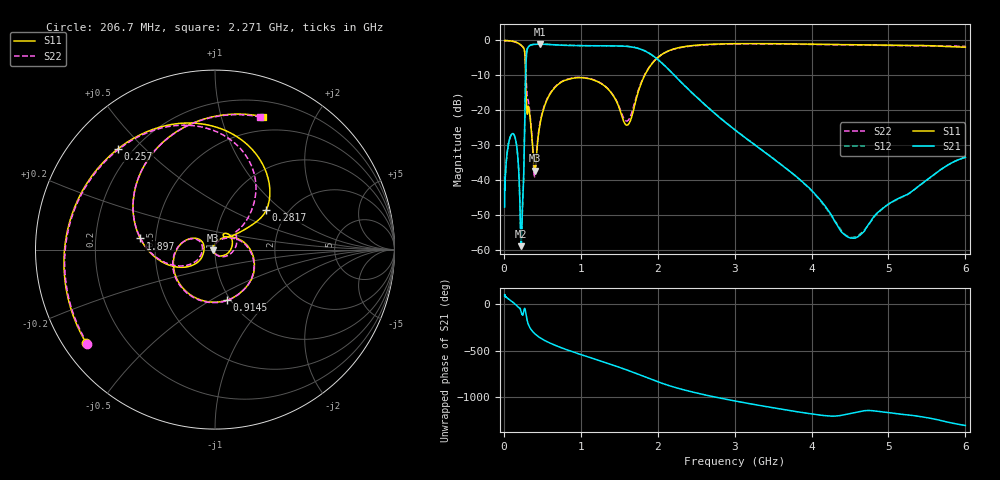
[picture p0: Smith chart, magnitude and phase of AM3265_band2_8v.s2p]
!Agilent Technologies,E8364B,MY43040894,A.07.50.67
!Agilent E8364B: A.07.50.67
!Date: Friday, May 09, 2025 07:26:20
!Correction: S11(Full 2 Port(1,2))
!S21(Full 2 Port(1,2))
!S12(Full 2 Port(1,2))
!S22(Full 2 Port(1,2))
!S2P File: Measurements: S11, S21, S12, S22:Log Frequency Sweep
# Hz S  dB  R 50
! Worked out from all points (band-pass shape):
!   3201 points, 10 MHz to 6 GHz, reference 50 ohm
!   highest |S21| = -1.08 dB at 465.3 MHz (marker M1); lowest = -59.0 dB at 226.6 MHz (marker M2)
!   |S21| within 3 dB of the highest: 294.5 MHz to 1.918 GHz (1.623 GHz wide, 147 % of centre)
!   lowest |S11| = -37.3 dB at 401.3 MHz (marker M3), VSWR 1.03, Z = 48.7 - j0.325 ohm
!   |S11| at or under -10 dB: 282.7 MHz to 1.831 GHz (1.549 GHz wide, 147 % of centre)
!   |S22| runs from -39.1 to 0.0 dB; largest |S21 - S12| = 0.0074
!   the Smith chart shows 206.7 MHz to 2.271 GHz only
!   S11 on the Smith chart (normalised r, x): 206.7 MHz: 0.07, -0.32; 257 MHz: 0.15, +0.42; 281.7 MHz: 1.56, +0.79; 914.5 MHz: 0.97, -0.59; 1.897 GHz: 0.41, +0.06; 2.271 GHz: 0.35, +1.36
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1e7  -0.07 -5.5  -47.80 85.3  -38.84 85.4  -0.10 -5.6
2.908064e7  -0.04 -15.8  -35.46 77.1  -35.35 76.8  -0.05 -15.8
8.439949e7  -0.12 -47.0  -27.61 42.0  -27.65 42.3  -0.16 -47.2
2.066717e8  -1.04 -143.9  -44.83 -44.1  -45.05 -43.1  -1.08 -143.5
2.265776e8  -1.39 -169.5  -59.00 -83.8  -56.66 -86.1  -1.42 -168.5
2.44949e8  -1.80 160.2  -45.95 -118.8  -45.90 -122.3  -1.81 162.5
2.569874e8  -2.17 133.8  -39.60 -83.9  -39.72 -84.5  -2.15 138.0
2.817395e8  -8.87 37.5  -11.12 -77.7  -11.09 -77.8  -7.00 59.7
3.113553e8  -19.68 59.6  -2.11 159.8  -2.08 159.8  -16.89 36.6
4.013416e8  -37.30 -165.9  -1.12 42.3  -1.09 42.3  -39.12 -178.0
4.653277e8  -24.59 68.0  -1.08 1.2  -1.05 1.2  -24.21 61.0
7.123273e8  -12.50 -22.0  -1.31 -98.3  -1.27 -98.3  -12.38 -25.5
9.145367e8  -10.76 -76.4  -1.47 -158.8  -1.43 -158.8  -10.67 -79.2
1.337069e9  -13.57 178.2  -1.54 85.6  -1.51 85.6  -13.51 178.0
1.897073e9  -7.51 171.5  -3.78 -84.1  -3.75 -84.0  -7.43 170.5
2.067357e9  -3.82 121.7  -6.74 -136.0  -6.72 -136.0  -3.84 122.0
2.271013e9  -2.08 70.2  -11.22 171.4  -11.19 171.5  -2.15 71.1
3.202913e9  -0.90 -91.4  -28.98 6.0  -28.95 6.0  -0.98 -91.5
3.818953e9  -1.01 -178.2  -39.35 -80.8  -39.37 -80.9  -1.09 -179.7
4.499191e9  -1.22 90.8  -56.63 -99.2  -56.48 -96.3  -1.31 89.3
5.195685e9  -1.41 -0.2  -44.66 -109.7  -44.71 -109.6  -1.52 -0.1
6e9  -1.93 -96.8  -33.54 132.2  -33.49 132.1  -1.68 -96.5
